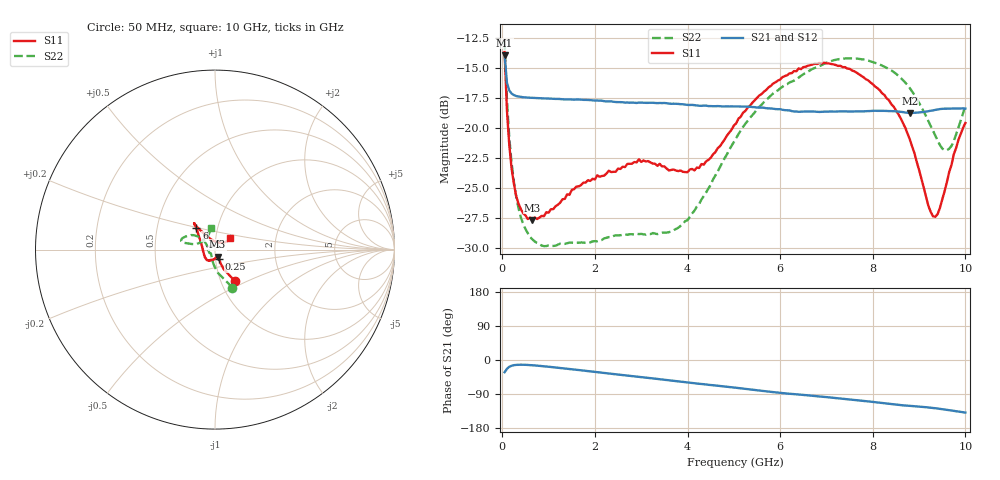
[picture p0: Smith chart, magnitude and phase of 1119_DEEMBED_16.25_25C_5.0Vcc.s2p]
!Hittite Microwave Corp.
!Digital Attenuator/PhaseShifter Rev 1.4.0
!Filename: C:\DATA\DATA\1119_DEEMBED_16.25_25C_5.0Vcc.s2p
!VNA ID: Agilent Technologies,N5224A,MY51441122,A.10.45.03
!Device type:
!2 Port Calibration.
!Temp(C): 25
!Lot Number:
!Serial Number:
!Operator:
!Misc:
!Attenuator:  16.250
# GHZ S DB R 50.0
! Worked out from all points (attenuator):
!   200 points, 50 MHz to 10 GHz, reference 50 ohm
!   highest |S21| = -13.89 dB at 50 MHz (marker M1); lowest = -18.7 dB at 8.8 GHz (marker M2)
!   lowest |S11| = -27.7 dB at 650 MHz (marker M3), VSWR 1.09, Z = 51.3 - j3.98 ohm
!   |S11| at or under -10 dB: start of sweep to end of sweep
!   |S22| runs from -29.9 to -12.7 dB; largest |S21 - S12| = 0.00034
!   S11 on the Smith chart (normalised r, x): 50 MHz: 1.17, -0.43; 250 MHz: 1.04, -0.11; 6 GHz: 0.79, +0.20; 10 GHz: 1.18, +0.15
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0.05  -13.64 -57.7  -13.89 -32.2  -13.89 -32.3  -12.67 -65.3
0.1  -18.51 -66.2  -16.20 -23.3  -16.20 -23.3  -17.61 -82.6
0.15  -21.38 -67.7  -16.85 -18.0  -16.85 -18.0  -20.75 -92.3
0.25  -24.65 -66.2  -17.24 -13.7  -17.25 -13.7  -24.49 -104.7
0.4  -26.77 -65.7  -17.39 -12.4  -17.40 -12.4  -27.46 -116.8
0.65  -27.69 -69.8  -17.47 -13.8  -17.47 -13.8  -29.31 -128.1
1.75  -24.57 -103.7  -17.64 -27.9  -17.64 -27.9  -29.58 -137.8
2.95  -22.61 -127.2  -17.87 -44.2  -17.88 -44.3  -28.87 -156.9
3.4  -22.99 -143.5  -17.90 -50.7  -17.91 -50.8  -28.82 -170.2
3.8  -23.60 -160.7  -17.98 -56.6  -17.99 -56.7  -28.34 174.1
4.25  -23.34 177.4  -18.13 -62.7  -18.14 -62.8  -26.36 155.4
5.05  -19.61 144.5  -18.19 -73.3  -18.20 -73.3  -20.83 140.6
6  -15.94 130.3  -18.42 -86.8  -18.44 -86.8  -16.68 146.8
6.7  -14.68 128.8  -18.61 -94.5  -18.62 -94.5  -15.05 155.0
7.5  -15.04 129.2  -18.61 -104.2  -18.62 -104.2  -14.17 164.0
8.35  -17.68 126.5  -18.58 -115.5  -18.58 -115.5  -15.06 167.4
8.8  -20.95 121.2  -18.73 -121.1  -18.72 -121.1  -16.66 167.1
9.2  -26.50 95.5  -18.59 -125.2  -18.60 -125.3  -19.42 162.7
9.35  -27.42 70.9  -18.48 -127.3  -18.50 -127.3  -20.64 155.7
9.5  -25.97 49.4  -18.39 -129.8  -18.41 -129.8  -21.71 143.1
9.65  -23.68 37.6  -18.37 -132.4  -18.39 -132.4  -21.73 126.5
10  -19.58 36.1  -18.37 -138.7  -18.37 -138.7  -18.09 99.5
